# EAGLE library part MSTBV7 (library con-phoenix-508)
PHOENIX
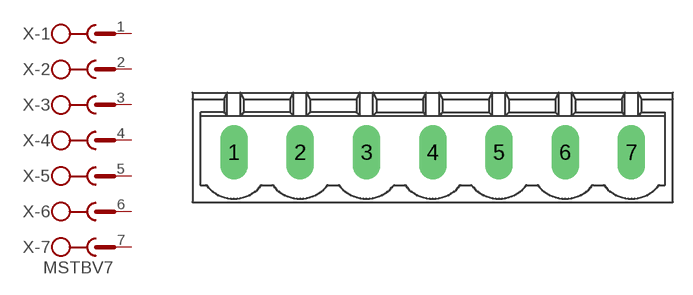
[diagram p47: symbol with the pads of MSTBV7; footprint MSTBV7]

Designator prefix X; gates -1=SK -2=SK -3=SK -4=SK -5=SK -6=SK -7=SKV

## MSTBV7 (OC_FARNELL: unknown; OC_NEWARK: unknown)  [MSTBV7]
1  -1:1  pas
2  -2:1  pas
3  -3:1  pas
4  -4:1  pas
5  -5:1  pas
6  -6:1  pas
7  -7:1  pas

## Footprint MSTBV7 (pad centres in mm)
PHOENIX
drill 1.397 long: 1 -15.24,0; 2 -10.16,0; 3 -5.08,0; 4 0,0; 5 5.08,0; 6 10.16,0; 7 15.24,0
